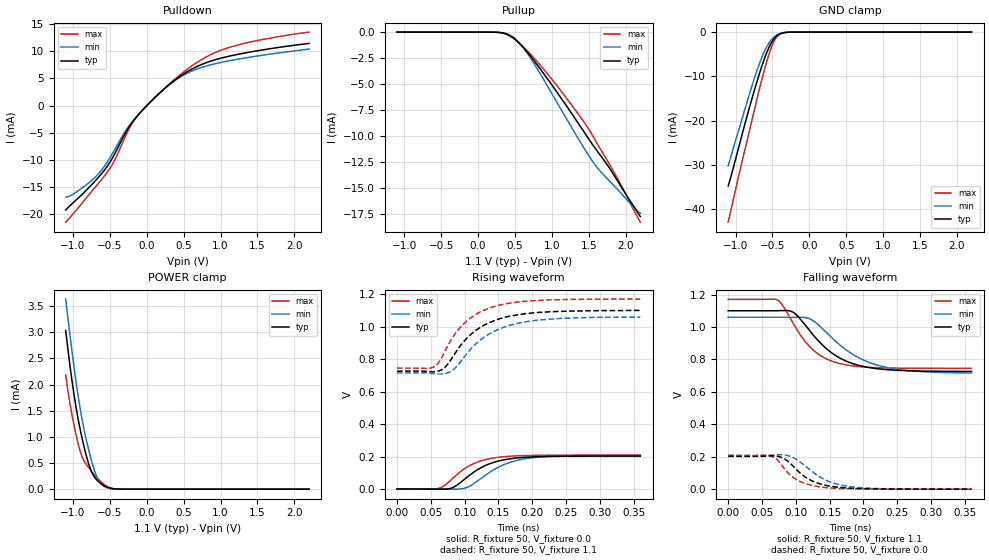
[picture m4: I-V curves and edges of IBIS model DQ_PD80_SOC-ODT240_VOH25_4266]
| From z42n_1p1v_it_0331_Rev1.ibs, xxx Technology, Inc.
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| DQ_PD80_SOC-ODT240_VOH25_4266
| (80 Ohm Pulldown, 240 Ohm System ODT Setting, VOH=VDDQ/2.5, 3200-4266Mbps)
[Model]   DQ_PD80_SOC-ODT240_VOH25_4266
Model_type   I/O
Vinl = 160.000mV
Vinh = 280.000mV
Vmeas = 220.000mV
Vref = 0.0mV
Cref = 0.0pF
Rref = 240.000Ohm
|   typ   min   max
|C_comp   0.834pF   0.784pF   0.884pF
C_comp_pullup   0.4170pF   0.3920pF   0.4420pF
C_comp_pulldown   0.4170pF   0.3920pF   0.4420pF
| Note: C_comp changes when the ODT circuit is enabled.
[Model Spec]
| Input threshold voltage corners
Vinl   0.1600V   0.1520V   0.1740V
Vinh   0.2800V   0.2720V   0.2940V
| Measurement voltage corners
Vmeas   0.2200V   0.2120V   0.2340V
| Timing spec test load voltage corners
Vref   0.0000V   0.0000V   0.0000V
| Dynamic Overshoot Parameters from LPDDR4 Specification
D_overshoot_ampl_h   0.30   NA   NA
D_overshoot_ampl_l   0.30   NA   NA
D_overshoot_area_h   0.1n   NA   NA
D_overshoot_area_l   0.1n   NA   NA
[Voltage Range]   1.1000V   1.0600V   1.1700V
[Pullup Reference]   1.1000V   1.0600V   1.1700V
| Junction Temperature (Ambient temp is 35C typ 95C min -40C max)
[Temperature Range]   50.0   110.0   -40.0
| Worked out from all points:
|   slope of the pulldown table from 0 to 0.165 V, typ, clamps not added: 74.4 ohm
|   slope of the pullup table from 0 to 0.165 V, typ, clamps not added: 53.4 kohm
|   GND clamp passes 1 mA (typ) near -0.45 V on its own axis
|   POWER clamp passes 1 mA (typ) near -0.88 V on its own axis
|   rising waveform, R_fixture 50, V_fixture 0.0: 20-80 % time 47.3ps typ, 51.4ps min, 43.6ps max; typ from 0 V to 0.203 V
|   falling waveform, R_fixture 50, V_fixture 1.1: 20-80 % time 57.2ps typ, 67.4ps min, 46.8ps max; typ from 1.1 V to 0.726 V
|   rising waveform, R_fixture 50, V_fixture 1.1: 20-80 % time 56.6ps typ, 59.8ps min, 51.9ps max; typ from 0.726 V to 1.1 V
|   falling waveform, R_fixture 50, V_fixture 0.0: 20-80 % time 38.9ps typ, 45.7ps min, 33.6ps max; typ from 0.203 V to 0 V
[Pulldown]
|   Voltage   I(typ)   I(min)   I(max)
-1.1V     -19.27mA   -16.9mA    -21.53mA
-918.5mV  -16.93mA   -15.62mA   -18.7mA
-654.5mV  -13.22mA   -12.57mA   -14.35mA
-469.7mV  -9.758mA   -8.945mA   -10.92mA
-275mV    -4.715mA   -4.422mA   -5.257mA
-139.7mV  -2.09mA    -2.067mA   -2.115mA
210.1mV   2.772mA    2.744mA    2.794mA
487.3mV   5.732mA    5.538mA    6.069mA
774.4mV   7.759mA    7.172mA    8.741mA
1.071V    8.972mA    8.141mA    10.52mA
1.58V     10.3mA     9.319mA    12.22mA
2.2V      11.48mA    10.44mA    13.57mA
[GND Clamp]
|   Voltage   I(typ)   I(min)   I(max)
-1.1V     -34.75mA   -30.21mA   -42.92mA
-944.9mV  -25.23mA   -21.44mA   -31.56mA
-796.4mV  -16.12mA   -13.14mA   -21.2mA
-727.1mV  -12.12mA   -9.512mA   -16.34mA
-661.1mV  -8.569mA   -6.433mA   -11.86mA
-588.5mV  -5.115mA   -3.68mA    -7.306mA
-522.5mV  -2.666mA   -1.902mA   -3.814mA
-469.7mV  -1.357mA   -988.9uA   -1.787mA
-413.6mV  -563.9uA   -417.7uA   -622.2uA
-350.9mV  -166.3uA   -126.6uA   -147.3uA
-235.4mV  -8.194uA   -7.718uA   -4.444uA
2.2V      0A         0A         0A
[Pullup]
|   Voltage   I(typ)   I(min)   I(max)
-1.1V     1.369uA    2.477uA    453.9nA
243.1mV   -14.42uA   -14.59uA   -13.76uA
388.3mV   -192.7uA   -160.4uA   -230.5uA
500.5mV   -687.6uA   -616.7uA   -720.8uA
602.8mV   -1.401mA   -1.397mA   -1.348mA
738.1mV   -2.555mA   -2.79mA    -2.331mA
1.085V    -5.922mA   -6.936mA   -5.288mA
1.448V    -9.706mA   -11.28mA   -8.764mA
1.655V    -11.81mA   -13.36mA   -11.2mA
1.887V    -14.24mA   -15.08mA   -14.02mA
2.094V    -16.57mA   -16.71mA   -16.87mA
2.2V      -17.73mA   -17.39mA   -18.26mA
[POWER Clamp]
|   Voltage   I(typ)   I(min)   I(max)
-1.1V     3.033mA    3.633mA    2.184mA
-1.041V   2.345mA    2.929mA    1.625mA
-981.2mV  1.753mA    2.275mA    1.183mA
-908.6mV  1.177mA    1.582mA    748.4uA
-852.5mV  818.5uA    1.148mA    543.7uA
-796.4mV  521.2uA    794.9uA    427.2uA
-740.3mV  306uA      494.5uA    324.2uA
-671mV    164.5uA    216uA      210.2uA
-598.4mV  83.68uA    71.96uA    113uA
-499.4mV  21.26uA    13.1uA     27.45uA
-387.2mV  1.88uA     1.297uA    1.61uA
2.2V      0A         0A         0A
[Ramp]
|   typ   min   max
| 20% - 80%
dV/dt_r   121.49m/47.34p   123.78m/51.42p   125.29m/43.58p
dV/dt_f   224.45m/57.19p   206.41m/67.38p   255.16m/46.73p
| 25% - 75%
|dV/dt_r   101.24m/37.61p   103.15m/41.00p   104.40m/34.62p
|dV/dt_f   187.04m/45.49p   172.01m/53.78p   212.63m/37.13p
R_load = 50
[Rising Waveform]
R_fixture = 50
V_fixture = 0.0
|   Time   V(typ)   V(min)   V(max)
0s        271.2uV    210uV      203.8uV
59ps      -359.1uV   126.2uV    1.346mV
69ps      -702uV     -544.8uV   18.12mV
79ps      3.718mV    -909uV     52.11mV
105ps     77.3mV     12.32mV    138.3mV
127ps     137.4mV    73.48mV    176.7mV
148ps     170.3mV    130.1mV    194.3mV
176ps     190.7mV    174.8mV    204mV
212ps     199.6mV    197.6mV    207.7mV
360ps     202.8mV    206.5mV    209mV
[Falling Waveform]
R_fixture   = 50
V_fixture   = 1.1
V_fixture_min = 1.06
V_fixture_max = 1.17
|   Time   V(typ)   V(min)   V(max)
0s        1.1V       1.06V      1.17V
73ps      1.1V       1.06V      1.166V
82ps      1.101V     1.06V      1.124V
97ps      1.088V     1.06V      1.016V
120ps     980.3mV    1.051V     881.1mV
140ps     886.5mV    987.6mV    814.9mV
163ps     813.3mV    896.7mV    776.5mV
192ps     764.4mV    812.5mV    756.3mV
229ps     738.9mV    755.6mV    748mV
360ps     725.9mV    716mV      744.7mV
[Rising Waveform]
R_fixture   = 50
V_fixture   = 1.1
V_fixture_min = 1.06
V_fixture_max = 1.17
|   Time   V(typ)   V(min)   V(max)
0s        725.5mV    714.2mV    744.7mV
56ps      722.4mV    710mV      755.3mV
63ps      728.3mV    708.1mV    786.7mV
72ps      754.1mV    711.4mV    857.2mV
83ps      816.6mV    734.5mV    937.7mV
96ps      894.2mV    793.8mV    1.006V
119ps     983.7mV    903mV      1.081V
147ps     1.042V     978mV      1.128V
217ps     1.09V      1.044V     1.163V
360ps     1.1V       1.059V     1.17V
[Falling Waveform]
R_fixture = 50
V_fixture = 0.0
|   Time   V(typ)   V(min)   V(max)
0s        202.9mV    206.6mV    209.1mV
59ps      205mV      208.1mV    208.6mV
76ps      199.9mV    212.6mV    166mV
88ps      173.1mV    207.8mV    102.1mV
99ps      129.4mV    188.1mV    64.35mV
116ps     69.44mV    136.4mV    31.98mV
135ps     33.73mV    77.08mV    14.66mV
160ps     13.18mV    32.16mV    5.437mV
192ps     4.137mV    10.48mV    1.627mV
360ps     352.2uV    347.4uV    229.3uV
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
